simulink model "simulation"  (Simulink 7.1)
settings: Solver=ode3  StartTime=0.0  StopTime=3  FixedStep=1e-4  MaxStep=1e  RelTol=1e-3
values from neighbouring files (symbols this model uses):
  b = 7.4272    [calculation.m]
  delta_1 = angle(EP)    [calculation.m]
  H = 3.5    [calculation.m]
  P_Peak_Fault = EP_Mag*VTH/XT_Fault,    [calculation.m]
  P_Peak_Post = EP_Mag*VB/XT_Post,    [calculation.m]
  Pm_PU = Pm/MVA_Base    (= 1)    [calculation.m]
  t_clear = 0.15    [calculation.m]
  Wsyn = 2*pi*60    (= 376.991118431)    [calculation.m]

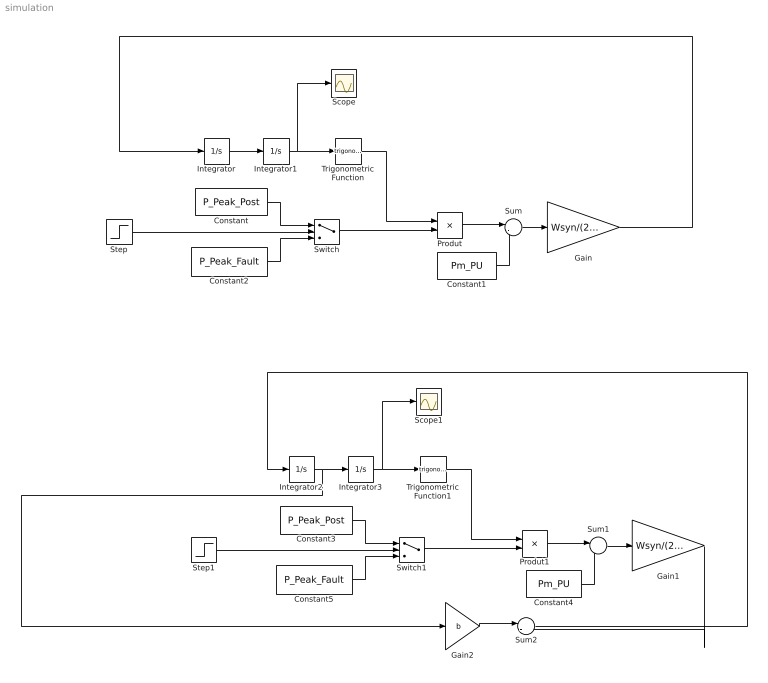
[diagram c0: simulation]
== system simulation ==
  Constant : Constant  Value=P_Peak_Post  OutDataType=sfix(16)  OutScaling=2^0
  Constant1 : Constant  Value=Pm_PU  OutDataType=sfix(16)  OutScaling=2^0
  Constant2 : Constant  Value=P_Peak_Fault  OutDataType=sfix(16)  OutScaling=2^0
  Constant3 : Constant  Value=P_Peak_Post  OutDataType=sfix(16)  OutScaling=2^0
  Constant4 : Constant  Value=Pm_PU  OutDataType=sfix(16)  OutScaling=2^0
  Constant5 : Constant  Value=P_Peak_Fault  OutDataType=sfix(16)  OutScaling=2^0
  Gain : Gain  Gain=Wsyn/(2*H)  ParameterDataType=sfix(16)  ParameterScaling=2^0  OutDataType=sfix(16)  OutScaling=2^0
  Gain1 : Gain  Gain=Wsyn/(2*H)  ParameterDataType=sfix(16)  ParameterScaling=2^0  OutDataType=sfix(16)  OutScaling=2^0
  Gain2 : Gain  Gain=b  ParameterDataType=sfix(16)  ParameterScaling=2^0  OutDataType=sfix(16)  OutScaling=2^0
  Integrator : Integrator
  Integrator1 : Integrator  InitialCondition=delta_1
  Integrator2 : Integrator
  Integrator3 : Integrator  InitialCondition=delta_1
  Produt : Product  OutDataType=sfix(16)  OutScaling=2^0
  Produt1 : Product  OutDataType=sfix(16)  OutScaling=2^0
  Scope : Scope
  Scope1 : Scope
  Step : Step  Time=t_clear  SampleTime=0
  Step1 : Step  Time=t_clear  SampleTime=0
  Sum : Sum  Inputs=|-+  OutDataType=sfix(16)  OutScaling=2^0
  Sum1 : Sum  Inputs=|-+  OutDataType=sfix(16)  OutScaling=2^0
  Sum2 : Sum  Inputs=|-+  OutDataType=sfix(16)  OutScaling=2^0
  Switch : Switch  Threshold=0.5
  Switch1 : Switch  Threshold=0.5
  Trigonometric Function : Trigonometry
  Trigonometric Function1 : Trigonometry
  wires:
  Integrator/1 -> Integrator1/1
  Integrator1/1 -> Trigonometric Function/1, Scope/1
  Trigonometric Function/1 -> Produt/1
  Constant1/1 -> Sum/2
  Produt/1 -> Sum/1
  Sum/1 -> Gain/1
  Gain/1 -> Integrator/1
  Switch/1 -> Produt/2
  Constant/1 -> Switch/1
  Constant2/1 -> Switch/3
  Step/1 -> Switch/2
  Integrator2/1 -> Integrator3/1, Gain2/1
  Integrator3/1 -> Trigonometric Function1/1, Scope1/1
  Trigonometric Function1/1 -> Produt1/1
  Constant4/1 -> Sum1/2
  Produt1/1 -> Sum1/1
  Sum1/1 -> Gain1/1
  Gain2/1 -> Sum2/1
  Gain1/1 -> Sum2/2
  Sum2/1 -> Integrator2/1
  Switch1/1 -> Produt1/2
  Constant3/1 -> Switch1/1
  Constant5/1 -> Switch1/3
  Step1/1 -> Switch1/2
